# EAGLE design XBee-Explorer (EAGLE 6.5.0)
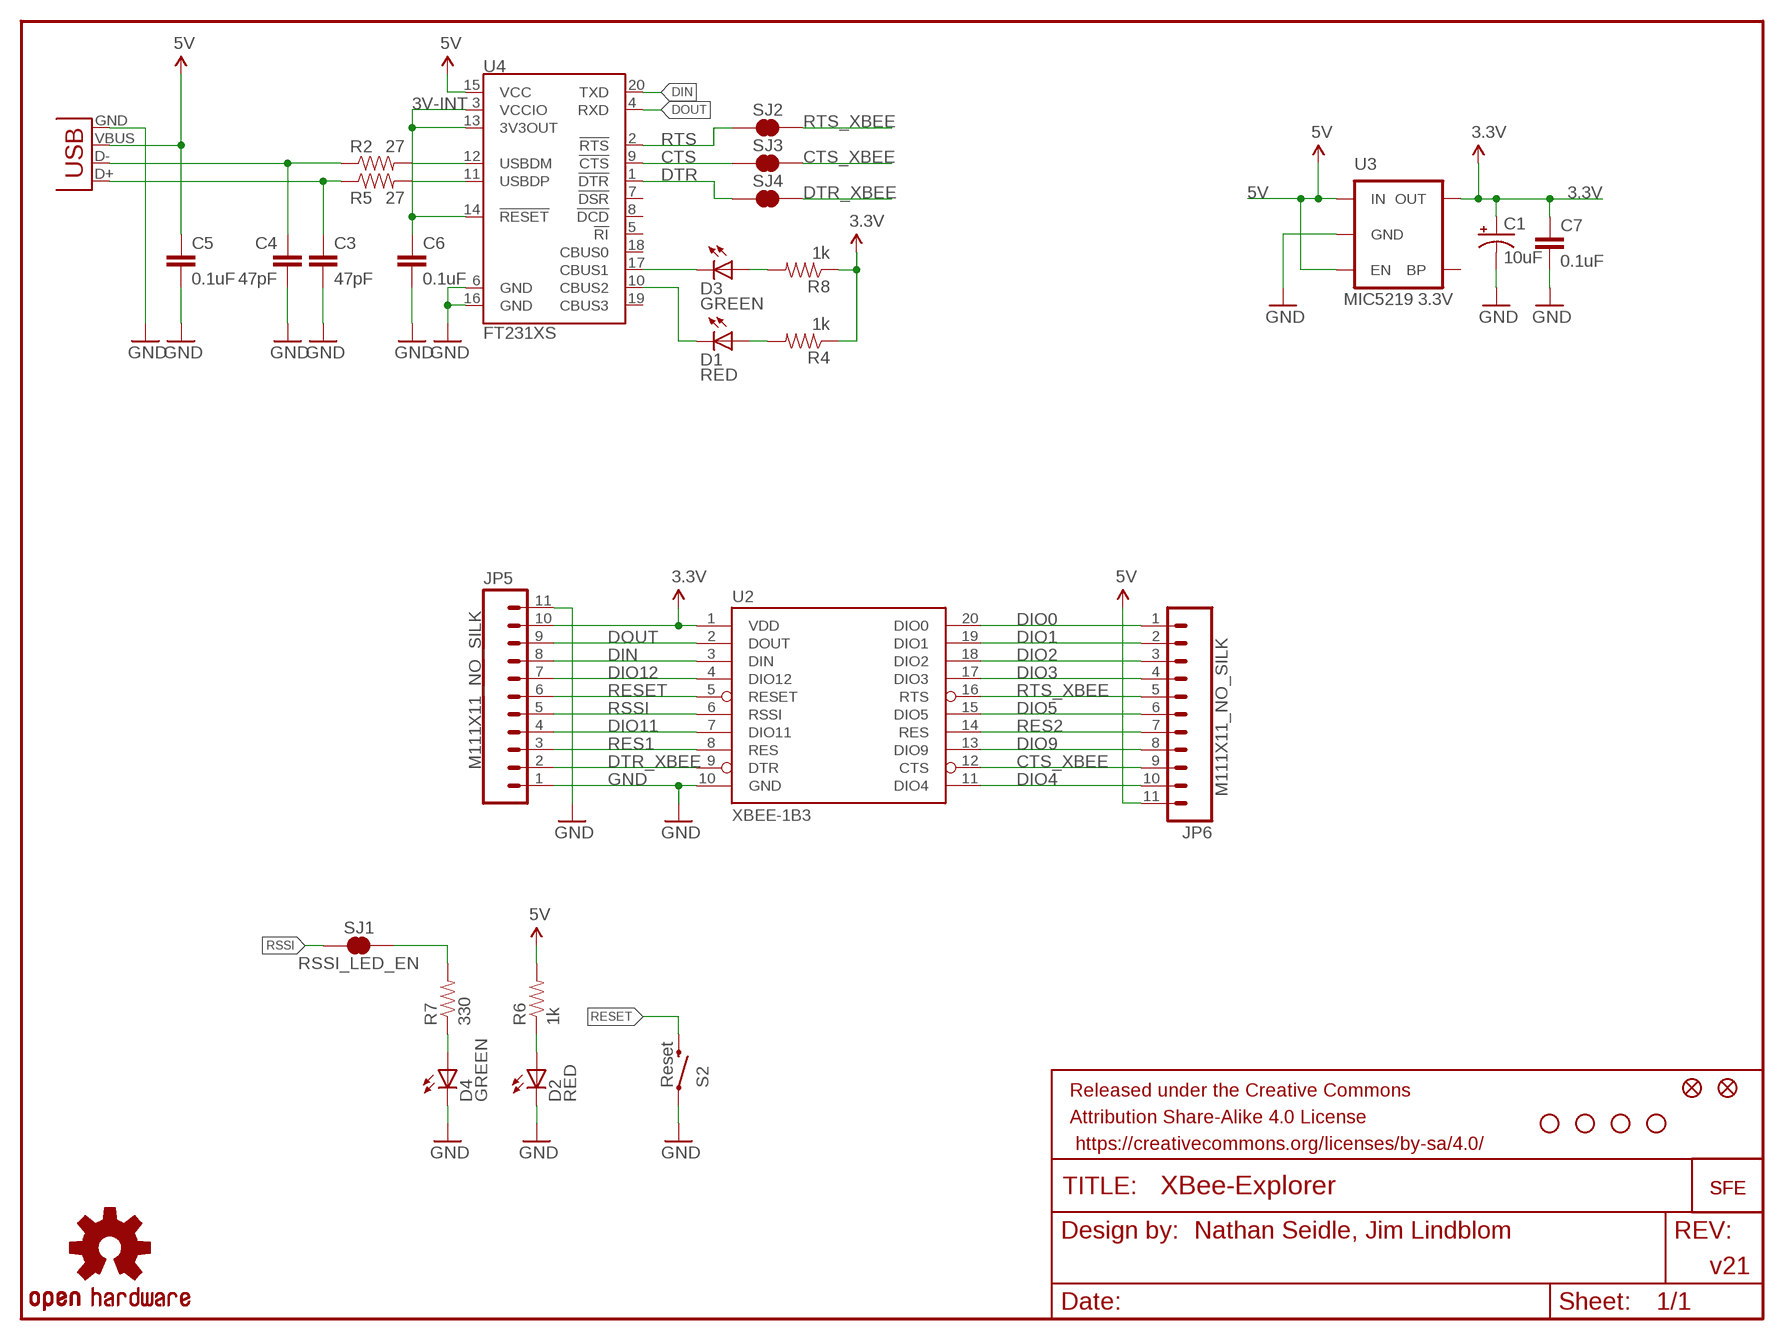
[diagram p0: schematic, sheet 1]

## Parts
C1  10uF  CAP_POL1206  [EIA3216]
C3  47pF  CAP0603-CAP  [0603-CAP]
C4  47pF  CAP0603-CAP  [0603-CAP]
C5  0.1uF  CAP0603-CAP  [0603-CAP]
C6  0.1uF  CAP0603-CAP  [0603-CAP]
C7  0.1uF  CAP0603-CAP  [0603-CAP]
D1  RED  LED-RED0603  [LED-0603]
D2  RED  LED-RED0603  [LED-0603]
D3  GREEN  LED-GREEN0603  [LED-0603]
D4  GREEN  LED-GREEN0603  [LED-0603]
FRAME1  FRAME-LETTER  [CREATIVE_COMMONS]
JP1  FIDUCIAL1X2  [FIDUCIAL-1X2]
JP4  FIDUCIAL1X2  [FIDUCIAL-1X2]
JP5  M111X11_NO_SILK  [1X11_NO_SILK]
JP6  M111X11_NO_SILK  [1X11_NO_SILK]
LOGO1  OSHW-LOGOS  [OSHW-LOGO-S]
R2  27  RESISTOR0603-RES  [0603-RES]
R4  1k  RESISTOR0603-RES  [0603-RES]
R5  27  RESISTOR0603-RES  [0603-RES]
R6  1k  RESISTOR0603-RES  [0603-RES]
R7  330  RESISTOR0603-RES  [0603-RES]
R8  1k  RESISTOR0603-RES  [0603-RES]
S2  Reset  SWITCH-MOMENTARY-2SMD  [TACTILE_SWITCH_SMD]
SJ1  RSSI_LED_EN  SOLDERJUMPERTRACE  [SJ_2S-TRACE]
SJ2  CTS_EN  SOLDERJUMPERTRACE  [SJ_2S-TRACE]
SJ3  RTS_EN  SOLDERJUMPERTRACE  [SJ_2S-TRACE]
SJ4  DTR  SOLDERJUMPERTRACE  [SJ_2S-TRACE]
U2  XBEE-1B3  [XBEE-SMD]
U3  MIC5219 3.3V  V_REG_LDOSMD  [SOT23-5]
U4  FT231XS  [SSOP20_L]
U$1  LOGO-SFESK  [SFE-LOGO-FLAME]
U$4  LOGO-SFENEW  [SFE-NEW-WEBLOGO]
U$5  STAND-OFF  [STAND-OFF]
U$9  STAND-OFF  [STAND-OFF]
U$10  STAND-OFF  [STAND-OFF]
U$11  STAND-OFF  [STAND-OFF]
X1  USBSMD  [USB-MINIB]

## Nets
3.3V: C1.A(+) C7.1 JP5.10 R4.1 R8.1 U2.1(VDD) U3.5(OUT)
3V-INT: C6.1 U4.3(VCCIO) U4.13(3V3OUT) U4.14(!RESET)
5V: C5.1 JP6.11 R6.2 U3.1(IN) U3.3(EN) U4.15(VCC) X1.VBUS
CTS: SJ3.1 U4.9(!CTS)
CTS_XBEE: JP6.9 SJ3.2 U2.12(CTS)
DIN: JP5.8 U2.3(DIN) U4.20(TXD)
DIO0: JP6.1 U2.20(DIO0)
DIO1: JP6.2 U2.19(DIO1)
DIO2: JP6.3 U2.18(DIO2)
DIO3: JP6.4 U2.17(DIO3)
DIO4: JP6.10 U2.11(DIO4)
DIO5: JP6.6 U2.15(DIO5)
DIO9: JP6.8 U2.13(DIO9)
DIO11: JP5.4 U2.7(DIO11)
DIO12: JP5.7 U2.4(DIO12)
DOUT: JP5.9 U2.2(DOUT) U4.4(RXD)
DTR: SJ4.1 U4.1(!DTR)
DTR_XBEE: JP5.2 SJ4.2 U2.9(DTR)
GND: C1.C(-) C3.2 C4.2 C5.2 C6.2 C7.2 D2.C D4.C JP5.1 JP5.11 S2.1 U2.10(GND) U3.2(GND) U4.6(GND) U4.16(GND) X1.GND
N$1: D1.A R4.2
N$2: D4.A R7.1
N$3: C3.1 R5.1 X1.D+
N$4: D3.A R8.2
N$5: C4.1 R2.1 X1.D-
N$6: D3.C U4.17(CBUS1)
N$7: R5.2 U4.11(USBDP)
N$8: R2.2 U4.12(USBDM)
N$9: R7.2 SJ1.2
N$38: D2.A R6.1
RES1: JP5.3 U2.8(RES)
RES2: JP6.7 U2.14(RES)
RESET: JP5.6 S2.3 U2.5(RESET)
RSSI: JP5.5 SJ1.1 U2.6(RSSI)
RTS: SJ2.1 U4.2(!RTS)
RTS_XBEE: JP6.5 SJ2.2 U2.16(RTS)
TXLED: D1.C U4.10(CBUS2)
Unconnected: U3.4(BP) U4.5(!RI) U4.7(!DSR) U4.8(!DCD) U4.18(CBUS0) U4.19(CBUS3)

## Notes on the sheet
- Nathan Seidle, Jim Lindblom
- v21

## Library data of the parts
C1 = SparkFun:CAP_POL: Capacitor Polarized
C3-C7 = SparkFun-Capacitors:CAP: Capacitor
D1 D2 = SparkFun-LED:LED-RED: Assorted Red LEDs; PROD_ID: DIO-00819
D3 D4 = SparkFun-LED:LED-GREEN: Various green LEDs; PROD_ID: DIO-00821
FRAME1 = SparkFun-Aesthetics:FRAME-LETTER: Schematic Frame
JP1 JP4 = SparkFun:FIDUCIAL: Fiducial Alignment Points
JP5 JP6 = SparkFun-Connectors:M11: Header 11 Standard 11-pin 0.1" header. Use with straight break away headers (SKU : PRT-00116), right angle break away headers (PRT-00553), swiss pins (PRT-00743), machine pins (PRT-00117), and female headers (PRT-00115).
LOGO1 = SparkFun-Aesthetics:OSHW-LOGO: Open Source Hardware Logo This logo indicates the piece of hardware it is found on incorporates a OSHW license and/or adheres to the definition of open source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
R2 R4-R8 = SparkFun-Resistors:RESISTOR: Resistor
S2 = SparkFun-Electromechanical:SWITCH-MOMENTARY-2: Various NO switches- pushbuttons, reed, etc; PROD_ID: SWCH-08247
SJ1-SJ4 = SparkFun-Passives:SOLDERJUMPER: Solder Jumper
U2 = SparkFun:XBEE-1
U3 = SparkFun:V_REG_LDO: Voltage Regulator LDO Standard 150mA LDO voltage regulator in SOT-23 layout. Micrel part MIC5205. BP (by-pass) pin is used to lower output noise with 470pF cap.
U4 = SparkFun-DigitalIC:FT231X: FTDI FT231X Full Speed USB to Full-handshake UART This USB2.0 Full Speed IC offers a compact bridge to full handshake UART interfaces. The device is a UART, capable of operating up to 3MBaud, with low power consumption (8mA). The FT231X includes the complete FT-X series feature set and enables USB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
U$1 U$4 = SparkFun:LOGO-SFE: Spark Fun Electronics PCB Logo
U$5 U$9-U$11 = SparkFun:STAND-OFF: Stand Off
X1 = SparkFun:USB: USB Connectors USB-B-PTH is fully proven SKU : PRT-00139 USB-miniB is fully proven SKU : PRT-00587 USB-A-PCB is untested. USB-A-H is throughly reviewed, but untested. Spark Fun Electronics SKU : PRT-00437 USB-B-SMT is throughly reviewed, but untested. Needs silkscreen touching up. USB-A-S has not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

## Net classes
0 default: width 0.203 mm
1 vcc: width 0.305 mm
2 gnd: width 0.254 mm

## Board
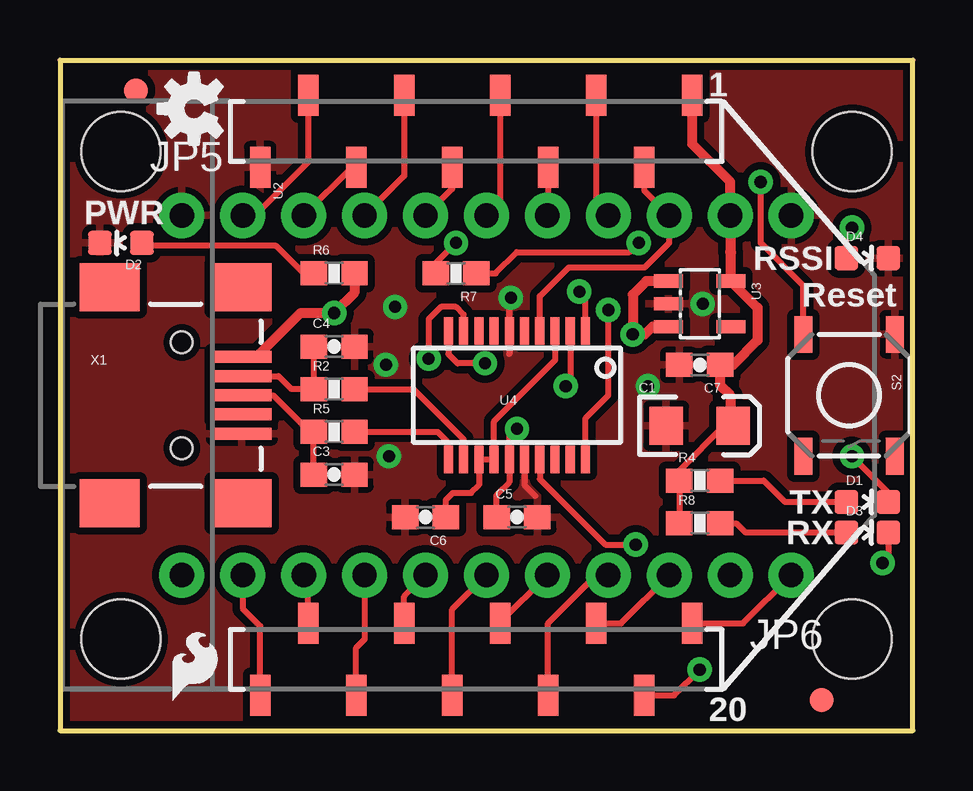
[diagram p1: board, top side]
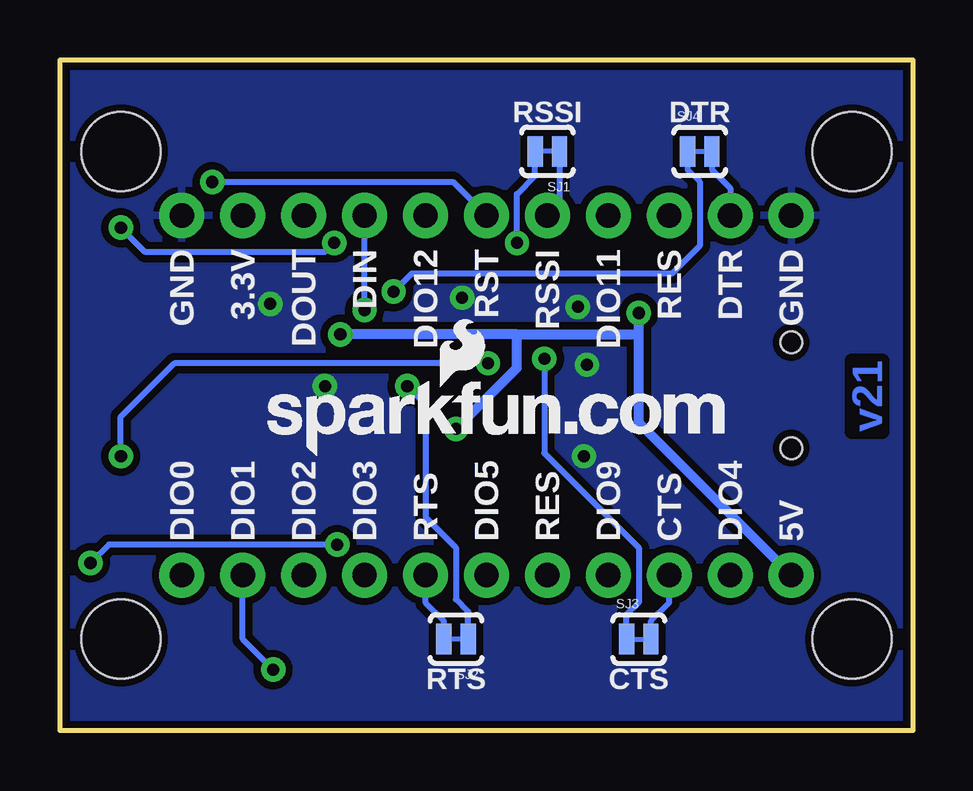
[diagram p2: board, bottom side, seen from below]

Size 35.56 x 27.94 mm. Coordinates in mm from the lower left corner, seen from the top.
Outline: 35.56,0 35.56,27.94 0,27.94 0,0 35.56,0
Copper layers (1*16): Top 0.035mm / dielectric 1.5mm / Bottom 0.035mm
Design rules "SparkFun-2-layer": minimum track width 7mil, minimum drill 15mil, track to track 8mil, track to pad 8mil, pad to pad 8mil, via to via 8mil, smd to smd 8mil, copper to edge 8mil, drill to drill 8mil, minimum pad ring 12mil, minimum via ring 10mil, stop-mask expansion 4mil, vias tented up to drill 20mil, thermal gap 10mil

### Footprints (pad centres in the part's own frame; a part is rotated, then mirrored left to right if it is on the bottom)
EIA3216 = smd 1.4 x 1.6: A 1.4,0; C -1.4,0
0603-CAP = smd 1.1 x 1: 1 -0.85,0; 2 0.85,0
LED-0603 = smd 1 x 1: A 0,-0.877; C 0,0.877
FIDUCIAL-1X2 = smd 1 x 1: 1 0,0
1X11_NO_SILK = drill 1.016 pad 1.88: 1 0,0; 2 2.54,0; 3 5.08,0; 4 7.62,0; 5 10.16,0; 6 12.7,0; 7 15.24,0; 8 17.78,0; 9 20.32,0; 10 22.86,0; 11 25.4,0
0603-RES = smd 1.1 x 1: 1 -0.85,0; 2 0.85,0
TACTILE_SWITCH_SMD = smd 1.524 x 0.762: 1 -2.54,1.905; 2 2.54,1.905; 3 -2.54,-1.905; 4 2.54,-1.905
SJ_2S-TRACE = smd 0.635 x 1.27: 1 -0.508,0; 2 0.508,0
XBEE-SMD = smd 1.7 x 0.85: 1 -12.5,20; 2 -9.5,18; 3 -12.5,16; 4 -9.5,14; 5 -12.5,12; 6 -9.5,10; 7 -12.5,8; 8 -9.5,6; 9 -12.5,4; 10 -9.5,2; 11 12.5,2; 12 9.5,4; 13 12.5,6; 14 9.5,8; 15 12.5,10; 16 9.5,12; 17 12.5,14; 18 9.5,16; 19 12.5,18; 20 9.5,20
SOT23-5 = smd 0.55 x 1.2: 1 -0.95,-1.3; 2 0,-1.3; 3 0.95,-1.3; 4 0.95,1.3; 5 -0.95,1.3
SSOP20_L = smd 0.381 x 1.143: 1 -2.857,-2.68; 2 -2.223,-2.68; 3 -1.587,-2.68; 4 -0.953,-2.68; 5 -0.318,-2.68; 6 0.318,-2.68; 7 0.953,-2.68; 8 1.587,-2.68; 9 2.223,-2.68; 10 2.857,-2.68; 11 2.857,2.68; 12 2.223,2.68; 13 1.587,2.68; 14 0.953,2.68; 15 0.318,2.68; 16 -0.318,2.68; 17 -0.953,2.68; 18 -1.587,2.68; 19 -2.223,2.68; 20 -2.857,2.68
STAND-OFF = hole 3.302: 0,0
USB-MINIB = smd 2.5 x 0.5: D+ 2.5,0; D- 2.5,0.8; GND 2.5,-1.6; ID 2.5,-0.8; VBUS 2.5,1.6 | smd 2.5 x 2: GND@1 -3,-4.5; GND@2 -3,4.5; GND@3 2.5,4.5; GND@4 2.5,-4.5 | hole 0.9: 0,2.2; 0,-2.2

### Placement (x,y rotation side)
C1  26.67,12.7 0 top
C3  11.43,10.67 0 top
C4  11.43,16 0 top
C5  19.05,8.89 0 top
C6  15.24,8.89 180 top
C7  26.67,15.24 180 top
D1  33.66,9.53 270 top
D2  2.54,20.32 90 top
D3  33.66,8.26 270 top
D4  33.66,19.68 270 top
FRAME1  not placed on the board
JP1  31.75,1.27 0 top
JP4  3.17,26.67 0 top
JP5  5.08,21.46 0 top
JP6  30.48,6.48 180 top
LOGO1  5.59,25.91 90 top
R2  11.43,14.22 0 top
R4  26.67,10.41 0 top
R5  11.43,12.45 0 top
R6  11.43,19.05 0 top
R7  16.51,19.05 180 top
R8  26.67,8.64 0 top
S2  32.89,13.97 270 top
SJ1  15.24,24.13 180 bottom
SJ2  19.05,3.81 180 bottom
SJ3  11.43,3.81 0 bottom
SJ4  8.89,24.13 0 bottom
U2  6.35,13.97 270 top
U3  26.67,17.78 270 top
U4  19.05,13.97 180 top
U$1  4.7,1.27 0 top
U$4  26.92,11.43 0 bottom
U$5  2.54,3.81 0 top
U$9  2.54,24.13 0 top
U$10  33.02,24.13 0 top
U$11  33.02,3.81 0 top
X1  5.08,13.97 0 top

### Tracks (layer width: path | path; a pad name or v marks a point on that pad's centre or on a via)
3.3V
  Top 0.254: R8.1 R4.1 25.82,10.83 27.69,12.7 C1.A
  Top 0.406: U2.1 26.35,24.45 27.94,22.86 JP5.10 27.94,19.94 27.97,19.91 U3.5 29.08,17.62 29.08,16.26 28.07,15.24 C7.1 27.52,14.39 27.94,13.97 27.94,12.83 C1.A
3V-INT
  Top 0.254: C6.1 16.09,9.61 16.38,9.91 17.14,9.91 17.46,10.22 U4.13 U4.14 18.1,12.89 20.64,15.43 U4.3
5V  (via drill 0.51)
  Top 0.254: v19.05,12.57 18.73,12.26 U4.15 18.73,10.35 18.2,9.82 C5.1
  Top 0.406: X1.VBUS 8.2,15.57 10.03,17.4 v11.43,17.4 12.28,18.25 R6.2 | U3.3 24.7,16.83 24.38,16.51 v23.88,16.51 23.88,18.16 24.45,18.73 U3.1
  Bottom 0.406: 16.51,16.51 v23.88,16.51 | v19.05,12.57 16.51,15.11 16.51,16.51 | 11.43,16.51 11.43,12.83 JP6.11 | 11.43,16.51 v11.43,17.4 | 16.51,16.51 11.43,16.51
CTS  (via drill 0.51)
  Top 0.254: U4.9 16.83,17.34 16.51,17.65 15.88,17.65 15.37,17.14 v15.37,15.49
  Bottom 0.254: v15.37,15.49 15.37,11.56 11.43,7.62 11.43,5.33 11.94,4.83 SJ3.1
CTS_XBEE
  Top 0.254: U2.12 10.35,6.29 JP6.9
  Bottom 0.254: SJ3.2 10.92,4.57 10.16,5.33 JP6.9
DIN  (via drill 0.51)
  Top 0.254: U2.3 22.35,21.97 JP5.8 | U4.20 21.91,13.02 22.86,13.97 v22.86,17.53
  Bottom 0.254: v22.86,17.53 JP5.8
DIO0
  Top 0.254: U2.20 28.47,4.47 JP6.1
DIO1  (via drill 0.51)
  Top 0.254: U2.19 25.6,1.47 v26.67,2.54
  Bottom 0.254: v26.67,2.54 27.94,3.81 JP6.2
DIO2
  Top 0.254: U2.18 23.39,4.47 JP6.3
DIO3
  Top 0.254: U2.17 20.35,4.47 22.35,6.48 JP6.4
DIO4
  Top 0.254: JP6.10 7.62,5.08 8.35,4.35 U2.11
DIO5
  Top 0.254: U2.15 16.35,5.05 JP6.6
DIO9
  Top 0.254: U2.13 12.35,3.46 12.7,3.81 JP6.8
DIO11
  Top 0.254: JP5.4 14.35,23.11 U2.7
DIO12
  Top 0.254: U2.4 20.35,21.49 JP5.7
DOUT
  Top 0.254: U2.2 24.35,22.51 JP5.9 25.4,20.32 24.38,19.3 21.21,19.3 20,18.1 U4.4
DTR  (via drill 0.51)
  Top 0.254: U4.1 21.91,18.03 v21.65,18.29
  Bottom 0.254: v21.65,18.29 20.89,19.05 10.03,19.05 8.89,20.19 8.89,22.86 9.4,23.37 SJ4.1
DTR_XBEE
  Top 0.254: JP5.2 8.13,21.46 10.35,23.68 U2.9
  Bottom 0.254: SJ4.2 8.38,23.37 7.62,22.61 JP5.2
GND  (via drill 0.51)
  Top 0.254: U4.16 19.37,10.22 19.81,9.78 | 18.73,15.68 U4.6 18.73,17.97 v18.8,18.03
  other vias: 24.51,14.35 13.72,11.43 13.59,15.24 26.8,17.78 13.97,17.65
  pour Bottom (isolate 0.305): 0,27.94 35.56,27.94 35.56,0 0,0
  pour Top (isolate 0.305): 0,27.94 35.56,27.94 35.56,0 0,0
N$1
  Top 0.254: R4.2 29.34,10.41 30.23,9.53 D1.A
N$2  (via drill 0.51)
  Top 0.254: R7.1 18.16,19.05 19.05,19.94 23.75,19.94 v24.13,20.32 | D4.A 32.78,20.71 v33.02,20.95
  Bottom 0.254: v24.13,20.32 24.51,19.94 32,19.94 v33.02,20.95
N$3
  Top 0.254: C3.1 R5.1 10.41,12.45 8.89,13.97 X1.D+
N$4
  Top 0.254: R8.2 28.19,8.64 28.57,8.26 D3.A
N$5
  Top 0.254: C4.1 R2.1 9.65,14.22 9.11,14.77 X1.D-
N$6  (via drill 0.51)
  Top 0.254: U4.17 20,10.48 22.73,7.75 v24,7.75 | D3.C 34.53,7.23 v34.29,6.99
  Bottom 0.254: v24,7.75 33.53,7.75 v34.29,6.99
N$7
  Top 0.254: R5.2 15.75,12.45 16.19,12 U4.11
N$8
  Top 0.254: R2.2 14.73,14.22 16.83,12.13 U4.12
N$9  (via drill 0.51)
  Top 0.254: R7.2 15.66,19.47 v16.51,20.32
  Bottom 0.254: v16.51,20.32 16.51,22.35 15.75,23.11 SJ1.2
N$38
  Top 0.254: R6.1 10.16,19.05 9.02,20.19 3.54,20.19 D2.A
RES1
  Top 0.254: JP5.3 12.17,23.47 U2.8
RES2
  Top 0.254: U2.14 14.35,5.59 JP6.7
RESET  (via drill 0.51)
  Top 0.254: U2.5 18.35,22.03 JP5.6 | S2.3 30.99,18.54 29.21,20.32 v29.21,22.86
  Bottom 0.254: v29.21,22.86 19.18,22.86 JP5.6
RSSI
  Top 0.254: U2.6 16.35,22.57 JP5.5
  Bottom 0.254: SJ1.1 14.73,21.97 JP5.5
RTS  (via drill 0.51)
  Top 0.254: U4.2 21.27,14.54 v21.08,14.35
  Bottom 0.254: v21.08,14.35 20.32,13.59 20.32,8.89 19.05,7.62 19.05,5.46 18.54,4.95 SJ2.1
RTS_XBEE
  Top 0.254: U2.16 18.35,4.51 JP6.5
  Bottom 0.254: SJ2.2 19.56,4.57 20.32,5.33 JP6.5
TXLED  (via drill 0.51)
  Top 0.254: U4.10 16.19,15.68 16.57,15.3 v17.72,15.3 | v33.02,11.43 34.53,9.92 D1.C
  Bottom 0.254: v17.72,15.3 30.8,15.3 33.02,13.08 v33.02,11.43

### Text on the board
Bottom: v21
tPlace: 1 | PWR | RSSI | Reset | TX | RX | 20
bPlace: DTR | RSSI | GND | DTR | RES | DIO11 | RSSI | RST | DIO12 | DIN | DOUT | 3.3V | GND | 5V | DIO4 | CTS | DIO9 | RES | DIO5 | RTS | DIO3 | DIO2 | DIO1 | DIO0 | CTS | RTS
tValues: XBee Socket Up | DNP | DNP | XBee Socket Up | N. Seidle
tDocu: Nathan Seidle, Jim Lindblom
